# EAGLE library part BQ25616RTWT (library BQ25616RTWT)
Battery Management Standalone 1-cell 3.0-A buck battery charger with power path and 1.2-A boost operation 24-WQFN -40 to 85 Source: Datasheet
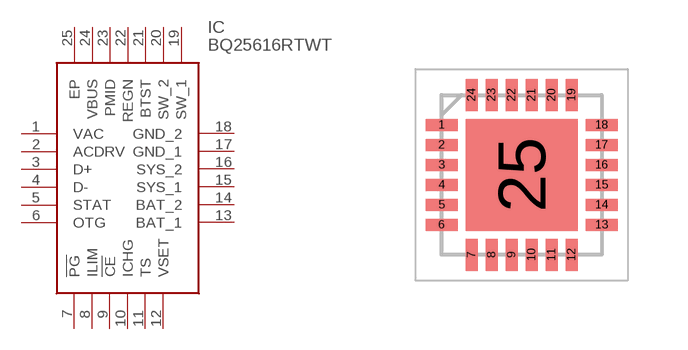
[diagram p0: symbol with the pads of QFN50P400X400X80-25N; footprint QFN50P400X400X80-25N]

Designator prefix IC

## BQ25616RTWT (Description: Battery Management Standalone 1-cell 3.0-A buck battery charger with power path and 1.2-A boost operation 24-WQFN -40 to 85; Height: 0.8mm; Manufacturer_Name: Texas Instruments; Manufacturer_Part_Number: BQ25616RTWT; Mouser_Part_Number: 595-BQ25616RTWT; Mouser_Price-Stock: https://www.mouser.co.uk/ProductDetail/Texas-Instruments/BQ25616RTWT?qs=GBLSl2AkirsF1eaqdbkEeA%3D%3D)  [QFN50P400X400X80-25N]
1  VAC
2  ACDRV
3  D+
4  D-
5  STAT
6  OTG
7  !PG
8  ILIM
9  !CE
10  ICHG
11  TS
12  VSET
13  BAT_1
14  BAT_2
15  SYS_1
16  SYS_2
17  GND_1
18  GND_2
19  SW_1
20  SW_2
21  BTST
22  REGN
23  PMID
24  VBUS
25  EP

## Footprint QFN50P400X400X80-25N (pad centres in mm)
RTW (S-PWQFN-N24)
smd 0.8 x 0.3: 1 -2,1.25; 2 -2,0.75; 3 -2,0.25; 4 -2,-0.25; 5 -2,-0.75; 6 -2,-1.25; 13 2,-1.25; 14 2,-0.75; 15 2,-0.25; 16 2,0.25; 17 2,0.75; 18 2,1.25
smd 0.3 x 0.8: 7 -1.25,-2; 8 -0.75,-2; 9 -0.25,-2; 10 0.25,-2; 11 0.75,-2; 12 1.25,-2; 19 1.25,2; 20 0.75,2; 21 0.25,2; 22 -0.25,2; 23 -0.75,2; 24 -1.25,2
smd 2.8 x 2.8: 25 0,0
